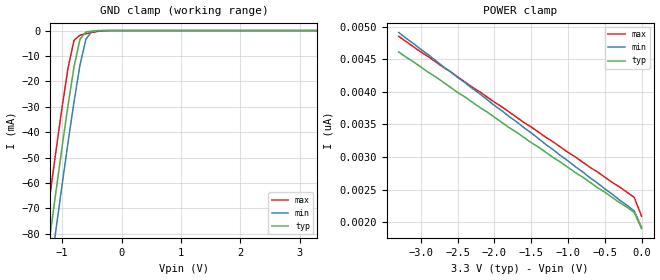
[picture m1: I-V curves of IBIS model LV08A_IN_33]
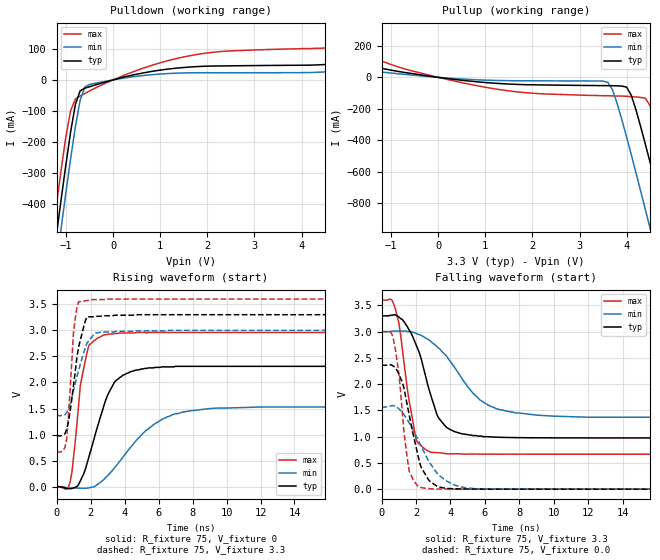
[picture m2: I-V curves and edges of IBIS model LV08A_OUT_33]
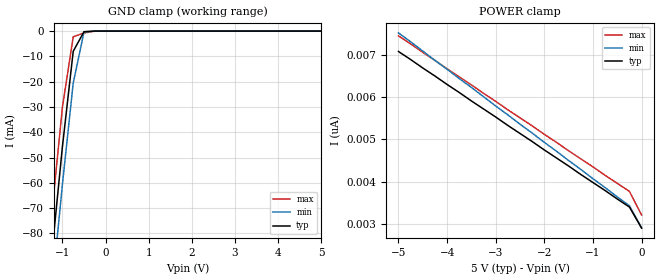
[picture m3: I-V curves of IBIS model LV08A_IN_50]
| TEXAS INSTRUMENTS INCORPORATED
| Standard Linear and Logic Group
| IBIS Model of SN74LV08A
| QUADRUPLE 2-INPUT POSITIVE-AND GATE
| SOIC 14-pin (D), SOP 14-pin (NS), SSOP 14-pin (DB), TSSOP 14-pin (PW)
| and TVSOP 14-pin (DGV) Package
[IBIS Ver]   3.2
[Comment Char]  |_char
[File Name]   lv08a.ibs
[File Rev]   2.0 I_die
[Date]   May 26, 2000
[Source]   Data created from HSPICE simulations at TI-SLL.
[Notes]   The following is an IBIS list for the LV08A.
|   Please contact sllibis@ti.com with questions and
|   comments concerning SLL IBIS models.
|   The warning about AC Rising Endpoint might be reported,
|   but it is due to HSPICE issue and negligible.
[Disclaimer] Property of Texas Instruments Incorporated.  Unauthorized
   reproduction and/or distribution is strictly prohibited.
   This product is protected under copyright law.
   Created 2000, (C) Copyright 2000, Texas Instruments Inc.,
   All Rights Reserved.
   UNLESS THERE IS A SIGNED, WRITTEN AGREEMENT TO THE
   CONTRARY, TEXAS INSTRUMENTS () IS PROVIDING THE IBIS
   MODELS  AND WITHOUT ANY WARRANTY, EXPRESSED OR
   IMPLIED.  TI assumes no liability for:
   1) the accuracy of the IBIS models provided to your
   company;
   2) the proper functioning of these IBIS Models in your
   design or for any resulting applications; or
   3) infringement of patents, copyrights or intellectual
   property rights resulting from your use of these IBIS
   models.
   TI provides IBIS Models as a service to our customers.
   You and your company shall not distribute, sell or give
   these models to anyone else without prior written
   permission from TI.
   TI reserves the right to make changes to our products or
   to discontinue any semiconductor product or service
   without notice, and advises our customers to obtain the
   latest version of relevant information to verify, before
   placing orders, that the information being relied on is
   current.
   Please be aware that your receipt and use of the IBIS
   information provided shall serve as acceptance of these
   terms and conditions.  If you do not accept these terms,
   you should return or destroy the IBIS models and any
   other accompanying information immediately.
|   Component LV08A_D
[Component]   LV08A_D
[Manufacturer]  Texas Instruments, Inc.
[Package]
|   typ   min   max
R_pkg   0.031   0.028   0.034
L_pkg   3.109nH   2.462nH   3.889nH
C_pkg   0.473pF   0.363pF   0.628pF
[Pin]   signal_name   model_name   R_pin   L_pin   C_pin
1   1A   LV08A_IN   0.033   3.854nH   0.622pF
2   1B   LV08A_IN   0.032   3.188nH   0.473pF
3   1Y   LV08A_OUT   0.028   2.462nH   0.377pF
4   2A   LV08A_IN   0.031   2.596nH   0.363pF
5   2B   LV08A_IN   0.028   2.521nH   0.372pF
6   2Y   LV08A_OUT   0.034   3.250nH   0.476pF
7   GND   GND   0.034   3.889nH   0.628pF
8   3Y   LV08A_OUT   0.034   3.889nH   0.628pF
9   3A   LV08A_IN   0.034   3.250nH   0.476pF
10   3B   LV08A_IN   0.028   2.521nH   0.372pF
11   4Y   LV08A_OUT   0.031   2.596nH   0.364pF
12   4A   LV08A_IN   0.028   2.462nH   0.377pF
13   4B   LV08A_IN   0.032   3.188nH   0.473pF
14   VCC   POWER   0.033   3.854nH   0.622pF
|   Component LV08A_NS
[Component]   LV08A_NS
[Manufacturer]  Texas Instruments, Inc.
[Package]
|   typ   min   max
R_pkg   0.045   0.039   0.054
L_pkg   3.796nH   2.561nH   4.952nH
C_pkg   0.528pF   0.288pF   0.710pF
[Pin]   signal_name   model_name   R_pin   L_pin   C_pin
1   1A   LV08A_IN   0.047   4.867nH   0.706pF
2   1B   LV08A_IN   0.051   4.083nH   0.592pF
3   1Y   LV08A_OUT   0.041   2.915nH   0.376pF
4   2A   LV08A_IN   0.039   2.561nH   0.288pF
5   2B   LV08A_IN   0.041   3.101nH   0.430pF
6   2Y   LV08A_OUT   0.047   4.047nH   0.589pF
7   GND   GND   0.051   4.909nH   0.700pF
8   3Y   LV08A_OUT   0.045   4.784nH   0.694pF
9   3A   LV08A_IN   0.054   4.176nH   0.597pF
10   3B   LV08A_IN   0.039   3.287nH   0.449pF
11   4Y   LV08A_OUT   0.039   2.586nH   0.294pF
12   4A   LV08A_IN   0.040   2.802nH   0.371pF
13   4B   LV08A_IN   0.049   4.080nH   0.593pF
14   VCC   POWER   0.052   4.952nH   0.710pF
|   Component LV08A_DB
[Component]   LV08A_DB
[Manufacturer]  Texas Instruments, Inc.
[Package]
|   typ   min   max
R_pkg   0.044   0.041   0.046
L_pkg   3.551nH   3.258nH   3.927nH
C_pkg   0.402pF   0.360pF   0.421pF
[Pin]   signal_name   model_name   R_pin   L_pin   C_pin
1   1A   LV08A_IN   0.046   3.927nH   0.408pF
2   1B   LV08A_IN   0.044   3.587nH   0.421pF
3   1Y   LV08A_OUT   0.041   3.289nH   0.398pF
4   2A   LV08A_IN   0.042   3.258nH   0.360pF
5   2B   LV08A_IN   0.041   3.286nH   0.403pF
6   2Y   LV08A_OUT   0.044   3.586nH   0.421pF
7   GND   GND   0.046   3.927nH   0.408pF
8   3Y   LV08A_OUT   0.046   3.927nH   0.408pF
9   3A   LV08A_IN   0.044   3.586nH   0.421pF
10   3B   LV08A_IN   0.041   3.286nH   0.403pF
11   4Y   LV08A_OUT   0.043   3.258nH   0.360pF
12   4A   LV08A_IN   0.041   3.289nH   0.398pF
13   4B   LV08A_IN   0.044   3.587nH   0.421pF
14   VCC   POWER   0.046   3.927nH   0.408pF
|   Component LV08A_PW
[Component]   LV08A_PW
[Manufacturer]  Texas Instruments, Inc.
[Package]
|   typ   min   max
R_pkg   0.032   0.029   0.035
L_pkg   2.378nH   2.170nH   2.680nH
C_pkg   0.314pF   0.270pF   0.335pF
[Pin]   signal_name   model_name   R_pin   L_pin   C_pin
1   1A   LV08A_IN   0.033   2.618nH   0.330pF
2   1B   LV08A_IN   0.031   2.313nH   0.317pF
3   1Y   LV08A_OUT   0.030   2.310nH   0.314pF
4   2A   LV08A_IN   0.031   2.173nH   0.272pF
5   2B   LV08A_IN   0.030   2.204nH   0.309pF
6   2Y   LV08A_OUT   0.032   2.315nH   0.317pF
7   GND   GND   0.035   2.680nH   0.335pF
8   3Y   LV08A_OUT   0.033   2.640nH   0.333pF
9   3A   LV08A_IN   0.034   2.347nH   0.319pF
10   3B   LV08A_IN   0.029   2.277nH   0.313pF
11   4Y   LV08A_OUT   0.031   2.170nH   0.270pF
12   4A   LV08A_IN   0.031   2.244nH   0.311pF
13   4B   LV08A_IN   0.033   2.343nH   0.321pF
14   VCC   POWER   0.035   2.657nH   0.332pF
|   Component LV08A_DGV
[Component]   LV08A_DGV
[Manufacturer]  Texas Instruments, Inc.
[Package]
|   typ   min   max
R_pkg   0.035   0.020   0.045
L_pkg   2.499nH   2.077nH   2.966nH
C_pkg   0.361pF   0.305pF   0.416pF
[Pin]   signal_name   model_name   R_pin   L_pin   C_pin
1   1A   LV08A_IN   0.027   2.717nH   0.373pF
2   1B   LV08A_IN   0.037   2.434nH   0.398pF
3   1Y   LV08A_OUT   0.034   2.200nH   0.316pF
4   2A   LV08A_IN   0.020   2.077nH   0.309pF
5   2B   LV08A_IN   0.030   2.147nH   0.305pF
6   2Y   LV08A_OUT   0.042   2.580nH   0.408pF
7   GND   GND   0.039   2.921nH   0.385pF
8   3Y   LV08A_OUT   0.033   2.841nH   0.380pF
9   3A   LV08A_IN   0.042   2.611nH   0.410pF
10   3B   LV08A_IN   0.038   2.331nH   0.329pF
11   4Y   LV08A_OUT   0.026   2.223nH   0.319pF
12   4A   LV08A_IN   0.034   2.259nH   0.313pF
13   4B   LV08A_IN   0.045   2.681nH   0.416pF
14   VCC   POWER   0.042   2.966nH   0.386pF
[Model Selector]   LV08A_IN
LV08A_IN_33   3.3-V Vcc Input Model
LV08A_IN_50   5.0-V Vcc Input Model
[Model Selector]   LV08A_OUT
LV08A_OUT_33   3.3-V Vcc Output Model
LV08A_OUT_50   5.0-V Vcc Output Model
| Models and submodels in the file (4): LV08A_IN_33 (Input), LV08A_OUT_33 (Output), LV08A_IN_50 (Input), LV08A_OUT_50 (Output)
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|   Model LV08A_IN_33
[Model]   LV08A_IN_33
Model_type  Input
Polarity   Inverting
Vinl = 0.99
Vinh = 2.31
| variable   typ   min   max
C_comp   1.24pf   0.94pf   1.54pf
[Temperature Range]   25   85   -40
[Voltage Range]   3.3   3.0   3.6
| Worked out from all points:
|   GND clamp passes 1 mA (typ) near -0.61 V on its own axis
[GND Clamp]
|   Voltage   I(typ)   I(min)   I(max)
-3.3V     -460mA     -475mA     -445mA
-1.3V     -97.5mA    -113mA     -81.5mA
-1.2V     -79.9mA    -95mA      -63.9mA
-1.1V     -62.6mA    -77.6mA    -46.7mA
-1V       -45.6mA    -60.5mA    -30mA
-900mV    -29.2mA    -43.9mA    -14.6mA
-800mV    -14.3mA    -28mA      -3.81mA
-700mV    -3.42mA    -13.6mA    -1.78mA
-600mV    -581uA     -3.4mA     -1.25mA
-500mV    -233uA     -353uA     -759uA
-400mV    -58.1uA    -21.9uA    -324uA
3.3V      1.9nA      2.34nA     1.69nA
[POWER Clamp]
|   Voltage   I(typ)   I(min)   I(max)
-3.3V     4.61nA     4.91nA     4.85nA
-3V       4.38nA     4.65nA     4.61nA
-100mV    2.15nA     2.17nA     2.38nA
0V        1.9nA      1.92nA     2.09nA
|   Model LV08A_OUT_33
[Model]   LV08A_OUT_33
Model_type  Output
Polarity   Non-Inverting
Vmeas = 1.65v
Cref = 15pf
| variable   typ   min   max
C_comp   4.62pf   3.47pf   5.77pf
[Temperature Range]   25   85   -40
[Voltage Range]   3.3   3.0   3.6
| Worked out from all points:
|   slope of the pulldown table from 0 to 0.495 V, typ, clamps not added: 27.3 ohm
|   slope of the pullup table from 0 to 0.495 V, typ, clamps not added: 27.2 ohm
|   rising waveform, R_fixture 75, V_fixture 0: 20-80 % time 1.34ns typ, 2.6ns min, 652ps max; typ from 0 V to 2.31 V
|   falling waveform, R_fixture 75, V_fixture 3.3: 20-80 % time 1.3ns typ, 2.37ns min, 767ps max; typ from 3.3 V to 0.976 V
|   rising waveform, R_fixture 75, V_fixture 3.3: 20-80 % time 624ps typ, 807ps min, 340ps max; typ from 0.976 V to 3.3 V
|   falling waveform, R_fixture 75, V_fixture 0.0: 20-80 % time 923ps typ, 1.58ns min, 574ps max; typ from 2.36 V to 0 V
[Pulldown]
|   Voltage   I(typ)   I(min)   I(max)
-3.3V     -3.04A     -3.13A     -2.95A
-1.3V     -615mA     -707mA     -518mA
-1.2V     -498mA     -591mA     -401mA
-1.1V     -383mA     -475mA     -288mA
-900mV    -167mA     -253mA     -98.6mA
-800mV    -79.1mA    -151mA     -61.7mA
-700mV    -35.5mA    -66.4mA    -51.9mA
-600mV    -26.8mA    -23.2mA    -43.9mA
-500mV    -22mA      -14.7mA    -35.8mA
1.6V      41.2mA     22.8mA     77.1mA
4.7V      52.1mA     27.5mA     106mA
6.6V      86.8mA     47.3mA     166mA
[Pullup]
|   Voltage   I(typ)   I(min)   I(max)
-3.3V     166mA      91.1mA     311mA
600mV     -21.6mA    -12.3mA    -39.7mA
3.6V      -52.9mA    -31.5mA    -117mA
3.8V      -54.2mA    -168mA     -119mA
4V        -62.6mA    -381mA     -121mA
4.1V      -115mA     -494mA     -123mA
4.4V      -429mA     -845mA     -133mA
4.5V      -544mA     -964mA     -182mA
4.8V      -899mA     -1.32A     -505mA
4.9V      -1.02A     -1.44A     -622mA
5.2V      -1.38A     -1.81A     -981mA
6.6V      -3.09A     -3.52A     -2.69A
[Ramp]
| variable   typ   min   max
dV/dt_r   1.40E+00/1.34E-09   9.37E-01/2.69E-09   1.78E+00/5.88E-10
dV/dt_f   1.41E+00/1.30E-09   9.88E-01/2.40E-09   1.77E+00/7.47E-10
R_load = 75
[Rising Waveform]
R_fixture = 75
V_fixture = 0
|   Time   V(typ)   V(min)   V(max)
0s        0V         0V         0V
800ps     -37.8mV    -20.7mV    90.5mV
1.1ns     -8.55mV    -24.3mV    863mV
1.4ns     112mV      -27.4mV    1.94V
1.8ns     453mV      -27.3mV    2.58V
2.7ns     1.46V      115mV      2.9V
3.9ns     2.14V      565mV      2.95V
5.7ns     2.28V      1.19V      2.96V
7.5ns     2.31V      1.44V      2.96V
25ns      2.31V      1.53V      2.96V
[Falling Waveform]
R_fixture = 75
V_fixture = 3.3
V_fixture_min = 3.0
V_fixture_max = 3.6
|   Time   V(typ)   V(min)   V(max)
0s        3.3V       3V         3.6V
800ps     3.32V      3.01V      3.43V
1ns       3.28V      3.01V      3.17V
2ns       2.75V      2.97V      951mV
2.8ns     1.85V      2.83V      710mV
3.3ns     1.36V      2.69V      695mV
4ns       1.13V      2.43V      673mV
5.7ns     1.01V      1.7V       667mV
7.3ns     985mV      1.48V      667mV
25ns      976mV      1.37V      666mV
[Rising Waveform]
R_fixture = 75
V_fixture = 3.3
V_fixture_min = 3.0
V_fixture_max = 3.6
|   Time   V(typ)   V(min)   V(max)
0s        976mV      1.37V      666mV
400ps     989mV      1.37V      700mV
600ps     1.11V      1.43V      924mV
800ps     1.45V      1.6V       1.86V
1ns       1.95V      1.85V      2.97V
1.3ns     2.68V      2.24V      3.55V
1.8ns     3.26V      2.76V      3.57V
2.2ns     3.26V      2.93V      3.59V
2.8ns     3.28V      2.97V      3.59V
25ns      3.3V       3V         3.6V
[Falling Waveform]
R_fixture = 75
V_fixture = 0.0
|   Time   V(typ)   V(min)   V(max)
0s        2.36V      1.56V      3V
500ps     2.37V      1.58V      3V
700ps     2.34V      1.59V      2.83V
1ns       2.19V      1.53V      2.21V
1.2ns     2.04V      1.47V      1.47V
1.6ns     1.42V      1.26V      344mV
2.2ns     514mV      884mV      36mV
3.2ns     58.4mV     312mV      1.97mV
4.8ns     4.06mV     30.1mV     1.34mV
25ns      12uV       591nV      14.1uV
|   Model LV08A_IN_50
[Model]   LV08A_IN_50
Model_type  Input
Polarity   Inverting
Vinl = 1.5
Vinh = 3.5
| variable   typ   min   max
C_comp   1.24pf   0.94pf   1.54pf
[Temperature Range]   25   85   -40
[Voltage Range]   5.0   4.5   5.5
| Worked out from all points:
|   GND clamp passes 1 mA (typ) near -0.52 V on its own axis
[GND Clamp]
|   Voltage   I(typ)   I(min)   I(max)
-5V       -773mA     -786mA     -758mA
-1.5V     -133mA     -148mA     -117mA
-1.25V    -88.7mA    -104mA     -72.7mA
-1V       -45.6mA    -60.5mA    -30mA
-750mV    -7.99mA    -20.5mA    -2.23mA
-500mV    -233uA     -353uA     -759uA
-250mV    -2.63nA    -182nA     -26.9uA
5V        2.9nA      3.64nA     2.54nA
[POWER Clamp]
|   Voltage   I(typ)   I(min)   I(max)
-5V       7.08nA     7.52nA     7.45nA
-1.5V     4.37nA     4.5nA      4.73nA
-250mV    3.4nA      3.43nA     3.77nA
0V        2.9nA      2.91nA     3.21nA
